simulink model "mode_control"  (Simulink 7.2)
settings: Solver=FixedStepDiscrete  SolverMode=SingleTasking  StartTime=0  StopTime=50  FixedStep=0.001  RelTol=1e-3
PreLoadFcn:
  | mode_control_prm;
  | xlsreadsdo('nxtscanner.xls','mpt');
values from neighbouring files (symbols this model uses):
  ERROR_001_SOUND_FREQ = 880    [mode_control_prm.m]
  ERROR_002_SOUND_FREQ = 220    [mode_control_prm.m]
  ERROR_SOUND_DUR = 3000    [mode_control_prm.m]
  ERROR_SOUND_VOL = 20    [mode_control_prm.m]
undefined symbols (not defined in the file or in its folder): Enum, ScanModeEnum, sigbuilder_block
libraries: mode_control_verification_lib x1

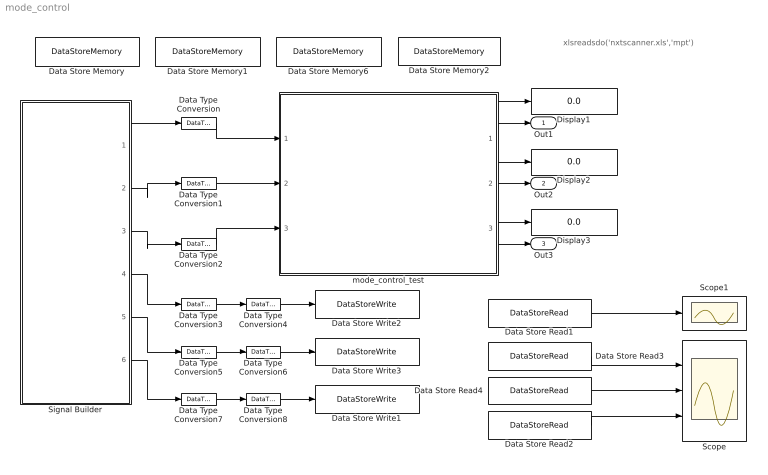
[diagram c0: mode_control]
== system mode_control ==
  note: xlsreadsdo('nxtscanner.xls','mpt')
  Data Store Memory : DataStoreMemory  DataStoreName=ControlMode  ReadBeforeWriteMsg=warning  WriteAfterWriteMsg=warning  WriteAfterReadMsg=warning  InitialValue=ControlModeEnum.INITIALIZE  DataType=Specify via dialog  OutDataType=Enum: ControlModeEnum  OutDataTypeStr=Enum: ControlModeEnum
  Data Store Memory1 : DataStoreMemory  DataStoreName=ErrorCode  ReadBeforeWriteMsg=warning  WriteAfterWriteMsg=warning  WriteAfterReadMsg=warning  InitialValue=ErrorCodeEnum.NO_ERROR  DataType=Specify via dialog  OutDataType=Enum: ErrorCodeEnum  OutDataTypeStr=Enum: ErrorCodeEnum
  Data Store Memory2 : DataStoreMemory  DataStoreName=FeedMode  ReadBeforeWriteMsg=warning  WriteAfterWriteMsg=warning  WriteAfterReadMsg=warning  InitialValue=FeedModeEnum.FEED_IDLE  DataType=Specify via dialog  OutDataType=Enum: FeedModeEnum  OutDataTypeStr=Enum: FeedModeEnum
  Data Store Memory6 : DataStoreMemory  DataStoreName=ScanMode  ReadBeforeWriteMsg=warning  WriteAfterWriteMsg=warning  WriteAfterReadMsg=warning  InitialValue=ScanModeEnum.SCAN_INIT  DataType=Specify via dialog  OutDataType=Enum: ScanModeEnum  OutDataTypeStr=Enum: ScanModeEnum
  Data Store Read1 : DataStoreRead  DataStoreName=ControlMode  SampleTime=-1
  Data Store Read2 : DataStoreRead  DataStoreName=ErrorCode  SampleTime=-1
  Data Store Read3 : DataStoreRead  DataStoreName=ScanMode  SampleTime=-1
  Data Store Read4 : DataStoreRead  DataStoreName=FeedMode  SampleTime=-1
  Data Store Write1 : DataStoreWrite  DataStoreName=ErrorCode  SampleTime=-1
  Data Store Write2 : DataStoreWrite  DataStoreName=ScanMode  SampleTime=-1
  Data Store Write3 : DataStoreWrite  DataStoreName=FeedMode  SampleTime=-1
  Data Type Conversion{,1..2,4,6,8} (6 alike) : DataTypeConversion  OutDataType=sfix(16)  OutScaling=2^0
  Data Type Conversion3 : DataTypeConversion  OutDataTypeMode=int8  OutDataType=sfix(16)  OutScaling=2^0  OutDataTypeStr=int8
  Data Type Conversion5 : DataTypeConversion  OutDataTypeMode=int8  OutDataType=sfix(16)  OutScaling=2^0  OutDataTypeStr=int8
  Data Type Conversion7 : DataTypeConversion  OutDataTypeMode=int8  OutDataType=sfix(16)  OutScaling=2^0  OutDataTypeStr=int8
  Display1 : Display
  Display2 : Display
  Display3 : Display
  Scope : Scope  NumInputPorts=3
  Scope1 : Scope
  Signal Builder : Subsystem  Tag=STV Subsys  LoadFcn=sigbuilder_block('load');  StartFcn=sigbuilder_block('start');  StopFcn=sigbuilder_block('stop');  ClipboardFcn=sigbuilder_block('clipboard');
  mode_control_test : Subsystem
  Out1 : Outport  OutDataType=sfix(16)  OutScaling=2^0
  Out2 : Outport  Port=2  OutDataType=sfix(16)  OutScaling=2^0
  Out3 : Outport  Port=3  OutDataType=sfix(16)  OutScaling=2^0
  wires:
  mode_control_test/1(Out1) -> Out1/1, Display1/1
  mode_control_test/2(Out2) -> Out2/1, Display2/1
  mode_control_test/3(Out3) -> Out3/1, Display3/1
  Data Type Conversion/1 -> mode_control_test/1(In1)
  Data Type Conversion1/1 -> mode_control_test/2(In2)
  Data Type Conversion2/1 -> mode_control_test/3(In3)
  Data Type Conversion3/1 -> Data Type Conversion4/1
  Data Type Conversion4/1 -> Data Store Write2/1
  Data Type Conversion5/1 -> Data Type Conversion6/1
  Data Type Conversion6/1 -> Data Store Write3/1
  Data Store Read1/1 -> Scope1/1
  Data Store Read3/1 -> Scope/1
  Data Store Read4/1 -> Scope/2
  Data Store Read2/1 -> Scope/3
  Data Type Conversion7/1 -> Data Type Conversion8/1
  Data Type Conversion8/1 -> Data Store Write1/1
  Signal Builder/2(PaperFeedBtn) -> Data Type Conversion1/1
  Signal Builder/3(ScanControlBtn) -> Data Type Conversion2/1
  Signal Builder/4(ScanMode) -> Data Type Conversion3/1
  Signal Builder/5(FeedMode) -> Data Type Conversion5/1
  Signal Builder/6(ErrorCode) -> Data Type Conversion7/1
  Signal Builder/1(PaperExhaustBtn) -> Data Type Conversion/1

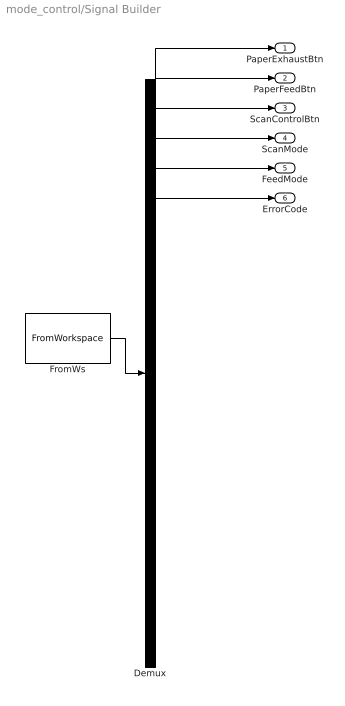
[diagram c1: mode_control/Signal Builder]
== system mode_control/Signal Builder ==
  Demux : Demux  Tag=STV Demux  Outputs=6
  FromWs : FromWorkspace  Tag=STV FromWs  VariableName=tuvar  SampleTime=0  SigBuilderData=DataTag0  VnvData=DataTag1
  PaperExhaustBtn : Outport  Tag=STV Outport
  PaperFeedBtn : Outport  Tag=STV Outport  Port=2
  ScanControlBtn : Outport  Tag=STV Outport  Port=3
  ScanMode : Outport  Tag=STV Outport  Port=4
  FeedMode : Outport  Tag=STV Outport  Port=5
  ErrorCode : Outport  Tag=STV Outport  Port=6
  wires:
  FromWs/1 -> Demux/1
  Demux/1 -> PaperExhaustBtn/1
  Demux/2 -> PaperFeedBtn/1
  Demux/3 -> ScanControlBtn/1
  Demux/4 -> ScanMode/1
  Demux/5 -> FeedMode/1
  Demux/6 -> ErrorCode/1

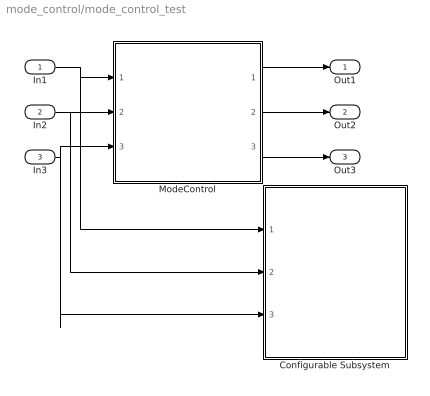
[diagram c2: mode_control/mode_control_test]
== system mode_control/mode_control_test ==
  In1 : Inport
  In2 : Inport  Port=2
  In3 : Inport  Port=3
  Configurable Subsystem : Subsystem  BlockChoice=Atomic Subsystem
  ModeControl : Subsystem  TreatAsAtomicUnit=on
  Out1 : Outport
  Out2 : Outport  Port=2
  Out3 : Outport  Port=3
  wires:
  In2/1 -> ModeControl/2(PaperFeedBtn), Configurable Subsystem/2(in1)
  ModeControl/1(SoundFreq) -> Out1/1
  In1/1 -> ModeControl/1(PaperExhaustBtn), Configurable Subsystem/1(in)
  ModeControl/2(SoundDur) -> Out2/1
  In3/1 -> ModeControl/3(ScanControlBtn), Configurable Subsystem/3(in2)
  ModeControl/3(SoundVol) -> Out3/1

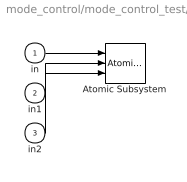
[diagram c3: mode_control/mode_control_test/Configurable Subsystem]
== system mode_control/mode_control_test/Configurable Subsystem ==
  in : Inport
  in1 : Inport  Port=2
  in2 : Inport  Port=3
  Atomic Subsystem : mode_control_verification_lib/Atomic Subsystem  SystemSampleTime=-1
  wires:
  in/1 -> Atomic Subsystem/1
  in1/1 -> Atomic Subsystem/2
  in2/1 -> Atomic Subsystem/3

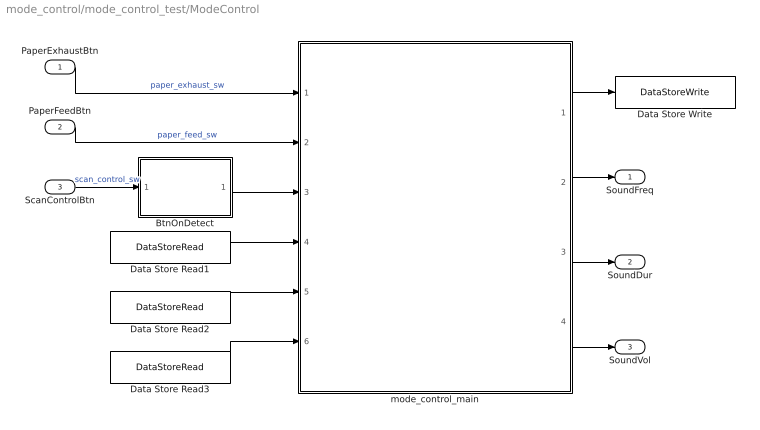
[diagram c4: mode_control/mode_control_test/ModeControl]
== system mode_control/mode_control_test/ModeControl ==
  PaperExhaustBtn : Inport
  PaperFeedBtn : Inport  Port=2
  ScanControlBtn : Inport  Port=3
  BtnOnDetect : Subsystem  TreatAsAtomicUnit=on
  Data Store Read1 : DataStoreRead  DataStoreName=ErrorCode  SampleTime=-1
  Data Store Read2 : DataStoreRead  DataStoreName=ScanMode  SampleTime=-1
  Data Store Read3 : DataStoreRead  DataStoreName=FeedMode  SampleTime=-1
  Data Store Write : DataStoreWrite  DataStoreName=ControlMode  SampleTime=-1
  mode_control_main : Stateflow chart
  SoundFreq : Outport  OutDataType=sfix(16)  OutScaling=2^0
  SoundDur : Outport  Port=2  OutDataType=sfix(16)  OutScaling=2^0
  SoundVol : Outport  Port=3  OutDataType=sfix(16)  OutScaling=2^0
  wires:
  mode_control_main/1(ControlMode) -> Data Store Write/1
  Data Store Read1/1 -> mode_control_main/4(ErrorCode)
  PaperFeedBtn/1 -> mode_control_main/2(PaperFeedBtn)  "paper_feed_sw"
  PaperExhaustBtn/1 -> mode_control_main/1(PaperExhaustBtn)  "paper_exhaust_sw"
  ScanControlBtn/1 -> BtnOnDetect/1(button)  "scan_control_sw"
  BtnOnDetect/1(off2on) -> mode_control_main/3(ScanControl)
  mode_control_main/2(SoundFreq) -> SoundFreq/1
  mode_control_main/3(SoundDur) -> SoundDur/1
  mode_control_main/4(SoundVol) -> SoundVol/1
  Data Store Read2/1 -> mode_control_main/5(ScanMode)
  Data Store Read3/1 -> mode_control_main/6(FeedMode)

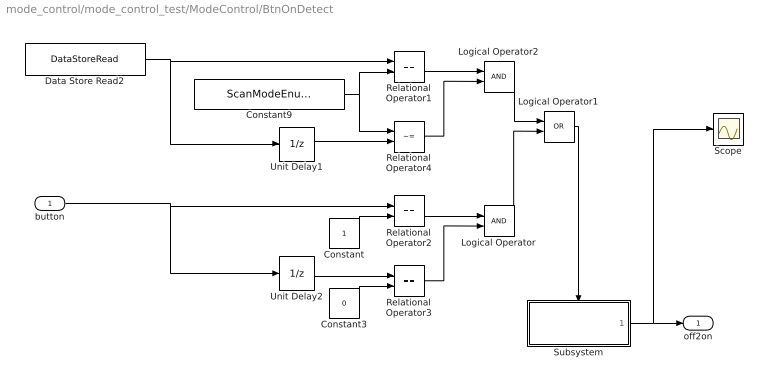
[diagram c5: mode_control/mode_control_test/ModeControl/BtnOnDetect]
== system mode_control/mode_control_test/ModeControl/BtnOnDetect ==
  button : Inport  OutDataType=sfix(16)  OutScaling=2^0
  Constant : Constant  OutDataTypeMode=uint8  OutDataType=sfix(16)  OutScaling=2^0  OutDataTypeStr=uint8
  Constant3 : Constant  Value=0  OutDataTypeMode=uint8  OutDataType=sfix(16)  OutScaling=2^0  OutDataTypeStr=uint8
  Constant9 : Constant  Value=ScanModeEnum.SCAN_INIT  OutDataTypeMode=Specify via dialog  OutDataType=Enum:ScanModeEnum  ConRadixGroup=Best Precision: Vector-wise  OutDataTypeStr=Enum:ScanModeEnum
  Data Store Read2 : DataStoreRead  DataStoreName=ScanMode  SampleTime=-1
  Logical Operator : Logic  AllPortsSameDT=off  OutDataTypeMode=boolean  OutDataTypeStr=boolean
  Logical Operator1 : Logic  Operator=OR  AllPortsSameDT=off  OutDataTypeMode=boolean  OutDataTypeStr=boolean
  Logical Operator2 : Logic  AllPortsSameDT=off  OutDataTypeMode=boolean  OutDataTypeStr=boolean
  Relational Operator1 : RelationalOperator  Operator===  LogicOutDataTypeMode=boolean  OutDataTypeStr=boolean
  Relational Operator2 : RelationalOperator  Operator===  LogicOutDataTypeMode=boolean  OutDataTypeStr=boolean
  Relational Operator3 : RelationalOperator  Operator===  LogicOutDataTypeMode=boolean  OutDataTypeStr=boolean
  Relational Operator4 : RelationalOperator  Operator=~=  LogicOutDataTypeMode=boolean  OutDataTypeStr=boolean
  Scope : Scope
  Subsystem : Subsystem  TreatAsAtomicUnit=on
  Unit Delay1 : UnitDelay  X0=ScanModeEnum.SCAN_INIT  SampleTime=-1
  Unit Delay2 : UnitDelay  SampleTime=-1
  off2on : Outport  OutDataType=sfix(16)  OutScaling=2^0
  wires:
  Relational Operator4/1 -> Logical Operator2/2
  Constant9/1 -> Relational Operator1/2, Relational Operator4/1
  Logical Operator2/1 -> Logical Operator1/1
  Relational Operator1/1 -> Logical Operator2/1
  Data Store Read2/1 -> Relational Operator1/1, Unit Delay1/1
  Logical Operator/1 -> Logical Operator1/2
  Logical Operator1/1 -> Subsystem/Enable
  Constant3/1 -> Relational Operator3/2
  Constant/1 -> Relational Operator2/2
  Relational Operator3/1 -> Logical Operator/2
  Relational Operator2/1 -> Logical Operator/1
  Unit Delay2/1 -> Relational Operator3/1
  button/1 -> Unit Delay2/1, Relational Operator2/1
  Unit Delay1/1 -> Relational Operator4/2
  Subsystem/1(Out1) -> Scope/1, off2on/1

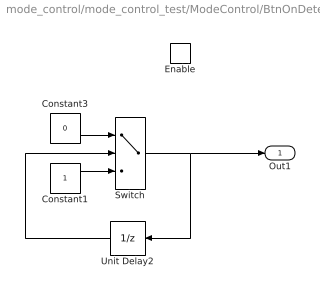
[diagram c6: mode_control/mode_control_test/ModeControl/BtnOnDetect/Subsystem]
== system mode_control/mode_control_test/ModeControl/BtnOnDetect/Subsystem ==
  Enable : EnablePort
  Constant1 : Constant  OutDataTypeMode=uint8  OutDataType=sfix(16)  OutScaling=2^0  OutDataTypeStr=uint8
  Constant3 : Constant  Value=0  OutDataTypeMode=uint8  OutDataType=sfix(16)  OutScaling=2^0  OutDataTypeStr=uint8
  Switch : Switch  Threshold=0.5
  Unit Delay2 : UnitDelay  Orientation=left  SampleTime=-1
  Out1 : Outport  OutDataType=sfix(16)  OutScaling=2^0
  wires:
  Switch/1 -> Out1/1, Unit Delay2/1
  Constant1/1 -> Switch/3
  Unit Delay2/1 -> Switch/2
  Constant3/1 -> Switch/1

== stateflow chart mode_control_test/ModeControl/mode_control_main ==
  state NORMAL/
    state IDLE/
      en:
      % no control
      ControlMode = IDLE;
    state PAPER_FEED/
      % paper feed button operation
      en:
      ControlMode = PAPERFEED;
    state PAPER_EXHAUST/
      % paper exhaust button operation
      en:
      ControlMode = PAPEREXHAUST;
    state SCAN_CONTROL/
      % scan control button operation
      en:
      ControlMode = SCAN;
    state INITIALIZE/
      en:
      % mecha initialize
      ControlMode = INITIALIZE;
    (default) -> INITIALIZE
    IDLE -> PAPER_FEED : [PaperFeedBtn == 1]
    PAPER_FEED -> IDLE : [PaperFeedBtn == 0]
    IDLE -> PAPER_EXHAUST : [PaperExhaustBtn == 1]
    PAPER_EXHAUST -> IDLE : [PaperExhaustBtn == 0]
    IDLE -> SCAN_CONTROL : [ScanControl == 1]
    SCAN_CONTROL -> INITIALIZE : [ScanControl == 0]
    INITIALIZE -> IDLE : [ScanMode == SCAN_IDLE && FeedMode == FEED_IDLE]
  state ERROR/
    % error job
    en:
    ControlMode = ERROR;
    % sound for system error
    SoundDur = ERROR_SOUND_DUR;
    SoundVol = ERROR_SOUND_VOL;
  NORMAL -> (junction 10) : [ErrorCode != NO_ERROR]
  (junction 10) -> (junction 11) : [ErrorCode == ERROR_001]
  (junction 11) -> (junction 12) : { % sound select SoundFreq = ERROR_001_SOUND_FREQ; }
  (junction 10) -> (junction 13) : { % sound select SoundFreq = ERROR_002_SOUND_FREQ; }
  (junction 12) -> (junction 13)
  (junction 13) -> ERROR
  (default) -> NORMAL
